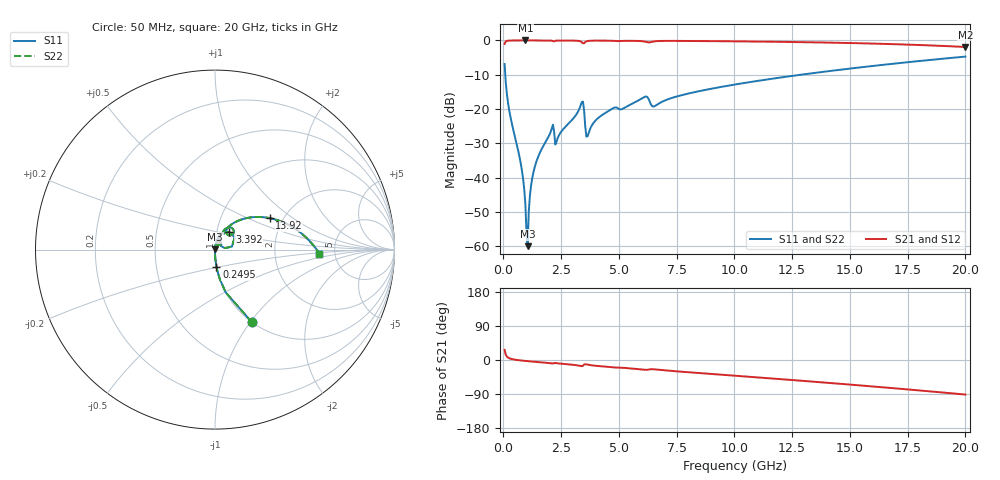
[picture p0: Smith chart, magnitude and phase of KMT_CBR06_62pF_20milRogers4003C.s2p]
! Data measured by Modelithics Inc. support@modelithics.com 813-866-6335
! KEMET CBR0603 62pF, Pad Width= 0.851mm, Pad Length= 0.64mm, Pad Gap= 0.62mm, 20mil Rogers 4003C substrate Data, January 2022
# hz S ma R 50
! 2 Port Network Data from SP1.SP block
! freq  magS11  angS11  magS21  angS21  magS12  angS12  magS22  angS22
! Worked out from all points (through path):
!   401 points, 50 MHz to 20 GHz, reference 50 ohm
!   highest |S21| = 0.00 dB at 947.8 MHz (marker M1); lowest = -1.9 dB at 20 GHz (marker M2)
!   group delay of S21, straight-line fit = 12.8 ps
!   lowest |S11| = -59.9 dB at 1.048 GHz (marker M3), VSWR 1.00, Z = 50.1 + j0.0868 ohm
!   |S11| at or under -10 dB: 79.36 MHz to 12.86 GHz (12.78 GHz wide, 198 % of centre)
!   |S22| runs from -59.9 to -4.7 dB; largest |S21 - S12| = 0
!   S11 on the Smith chart (normalised r, x): 50 MHz: 1.00, -1.02; 249.5 MHz: 1.00, -0.19; 3.392 GHz: 1.15, +0.23; 13.92 GHz: 1.70, +0.68; 20 GHz: 3.76, -0.25
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5e7  0.4541 -63.1  0.8906 26.9  0.8906 26.9  0.4541 -63.1
2.495e8  0.09601 -85.1  0.9951 4.8  0.9951 4.8  0.09601 -85.1
7.4825e8  0.01624 -89.8  0.9994 -1.2  0.9994 -1.2  0.01624 -89.8
8.48e8  0.009793 -89.4  0.9995 -1.9  0.9995 -1.9  0.009793 -89.4
9.4775e8  0.00418 -86.4  0.9995 -2.5  0.9995 -2.5  0.00418 -86.4
1.0475e9  0.001009 59.3  0.9995 -3.0  0.9995 -3.0  0.001009 59.3
1.097375e9  0.003291 78.3  0.9995 -3.3  0.9995 -3.3  0.003291 78.3
1.197125e9  0.007749 82.4  0.9994 -3.8  0.9994 -3.8  0.007749 82.4
1.296875e9  0.01197 83.1  0.9993 -4.4  0.9993 -4.4  0.01197 83.1
1.646e9  0.02586 82.3  0.9989 -6.2  0.9989 -6.2  0.02586 82.3
2.045e9  0.04662 77.1  0.9953 -8.5  0.9953 -8.5  0.04662 77.1
2.34425e9  0.03755 75.1  0.9952 -8.8  0.9952 -8.8  0.03755 75.1
3.391625e9  0.1261 50.6  0.9437 -16.3  0.9437 -16.3  0.1261 50.6
3.690875e9  0.0451 60.2  0.9858 -13.0  0.9858 -13.0  0.0451 60.2
4.73825e9  0.1026 66.4  0.9869 -19.3  0.9869 -19.3  0.1026 66.4
6.13475e9  0.152 53.0  0.9595 -26.0  0.9595 -26.0  0.152 53.0
6.73325e9  0.1208 58.7  0.9813 -26.0  0.9813 -26.0  0.1208 58.7
1.0025e10  0.2281 48.0  0.9709 -41.4  0.9709 -41.4  0.2281 48.0
1.336662e10  0.3329 32.6  0.9396 -56.9  0.9396 -56.9  0.3329 32.6
1.391525e10  0.3514 29.9  0.9326 -59.6  0.9326 -59.6  0.3514 29.9
1.670825e10  0.4518 15.9  0.8869 -73.5  0.8869 -73.5  0.4518 15.9
2e10  0.5816 -2.2  0.8027 -91.2  0.8027 -91.2  0.5816 -2.2
